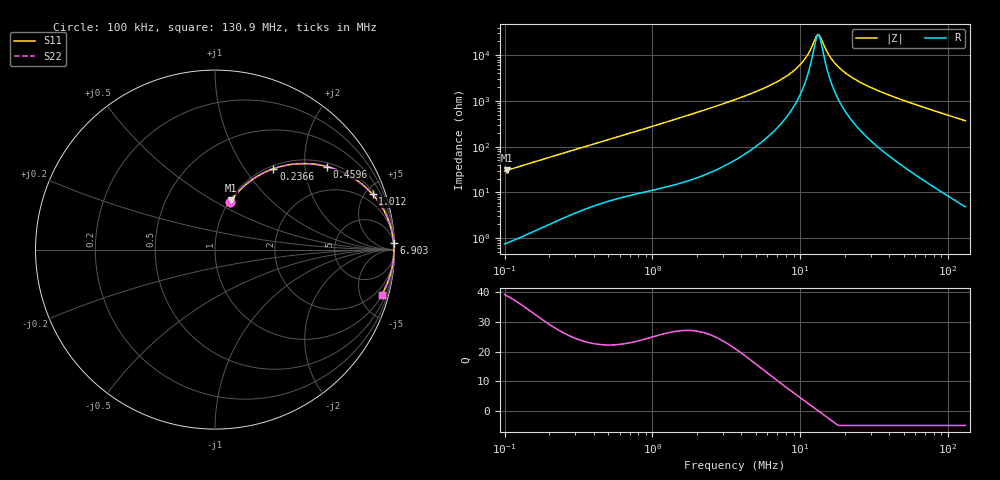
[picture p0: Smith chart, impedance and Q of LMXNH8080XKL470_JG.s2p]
! LMXNH8080XKL470_JG  S-PARAMETER MODEL  ( General Type )
! Model Generated by TAIYO YUDEN Corporation (http://www.ty-top.com)
! Version 1.0
! TAIYO YUDEN Control No. 191025NI43SB-FBB
! Copyright(c) 2019 TAIYO YUDEN CO.,LTD. All Rights Reserved.
! Product Description (link to TY-COMPAS)
! https://ds.yuden.co.jp/TYCOMPAS/or/detail?pn=LMXNH8080XKL470MJG&u=M
! Products Name : Inductors
! Characteristics :
!  Inductance : 47 uH , SRF(min) : 11 MHz , DC Resistance(max) : 0.221 Ohm
!  Rated Current : Saturation :1100 mA , Temp Rise : 1300 mA
!  Case Size : 8.0 x 8.0 / 0.315 x 0.315 [mm/inch] , Thickness : 3 / 0.118 [mm/inch]
!  (Conditions: Temperature = 25 degC , DC Bias Current/Voltage = 0A / 0V)
! External Node Assignments :
!  1  o---GGG---o  2
! GND o---------o GND
! Frequency Range : 0.1MHz  -  130.914307MHz  [ 402 STEP ]
# MHz S RI R 50
! Freq[MHz].  S11 Real  S11 Imag  S21 Real  S21 Imag  S12 Real  S12 Imag  S22 Real  S22 Imag
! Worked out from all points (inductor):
!   401 points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, 100 kHz to 130.9 MHz, reference 50 ohm
!   read as one part in series: L = 46.6 uH near 103.7 kHz
!   highest Q = 38.9 at 103.7 kHz (marker M1), where L = 46.7 uH
!   self-resonance near 13.17 MHz
!   S11 on the Smith chart (normalised r, x): 100 kHz: 1.01, +0.59; 236.6 kHz: 1.05, +1.37; 459.6 kHz: 1.12, +2.61; 1.012 MHz: 1.22, +5.62; 6.903 MHz: 6, +51; 130.9 MHz: 1.10, -7.35
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0.1  0.0851 0.2666  0.9149 -0.2666  0.9149 -0.2666  0.0851 0.2666
0.103654  0.0906 0.2744  0.9094 -0.2744  0.9094 -0.2744  0.0906 0.2744
0.156607  0.1805 0.3697  0.8195 -0.3697  0.8195 -0.3697  0.1805 0.3697
0.236613  0.3259 0.4505  0.6741 -0.4505  0.6741 -0.4505  0.3259 0.4505
0.332733  0.4779 0.4788  0.5221 -0.4788  0.5221 -0.4788  0.4779 0.4788
0.459579  0.6243 0.4624  0.3757 -0.4624  0.3757 -0.4624  0.6243 0.4624
0.682015  0.775 0.3963  0.225 -0.3963  0.225 -0.3963  0.775 0.3963
1.012111  0.8782 0.3077  0.1218 -0.3077  0.1218 -0.3077  0.8782 0.3077
1.10711  0.8952 0.2874  0.1048 -0.2874  0.1048 -0.2874  0.8952 0.2874
3.683715  0.9874 0.0902  0.0126 -0.0902  0.0126 -0.0902  0.9874 0.0902
6.902754  0.9948 0.0383  0.00519 -0.0383  0.00519 -0.0383  0.9948 0.0383
8.408907  0.9957 0.0258  0.00429 -0.0258  0.00429 -0.0258  0.9957 0.0258
9.706872  0.9961 0.0173  0.00388 -0.0173  0.00388 -0.0173  0.9961 0.0173
11.00592  0.9964 0.0102  0.00365 -0.0102  0.00365 -0.0102  0.9964 0.0102
12.03896  0.9964 0.00517  0.00355 -0.00517  0.00355 -0.00517  0.9964 0.00517
12.93477  0.9965 0.00121  0.00352 -0.00121  0.00352 -0.00121  0.9965 0.00121
13.40737  0.9965 -0.000769  0.00351 0.000769  0.00351 0.000769  0.9965 -0.000769
16.04237  0.9964 -0.0107  0.0036 0.0107  0.0036 0.0107  0.9964 -0.0107
19.19522  0.9961 -0.021  0.00392 0.021  0.00392 0.021  0.9961 -0.021
25.57835  0.995 -0.039  0.00499 0.039  0.00499 0.039  0.995 -0.039
40.05754  0.991 -0.074  0.00898 0.074  0.00898 0.074  0.991 -0.074
130.9143  0.9283 -0.2515  0.0717 0.2515  0.0717 0.2515  0.9283 -0.2515
